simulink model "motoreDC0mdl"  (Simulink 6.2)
settings: Solver=ode45  StartTime=0.0  StopTime=10.0  RelTol=1e-6  AbsTol=1e-6
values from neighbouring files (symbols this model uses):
  bme = Ic0*KI/Wmax    (= 1.40697764938e-05)    [motoreDC0.m]
  Ime0 = 0    [motoreDC0.m]
  Jme = 7.06*mg*m^2    (= 7.06e-06)    [motoreDC0.m]
  KI = Cmax/Imax    (= 0.0452697095436)    [motoreDC0.m]
  Lme = 2.63*mHenry    (= 0.00263)    [motoreDC0.m]
  Rme0 = Vn/Imax    (= 2.48962655602)    [motoreDC0.m]
  Tcsim = 1*msec    (= 0.001)    [motoreDC0.m]
  th0 = 0    [motoreDC0.m]
  Wme0 = 0    [motoreDC0.m]
libraries: simulink x2

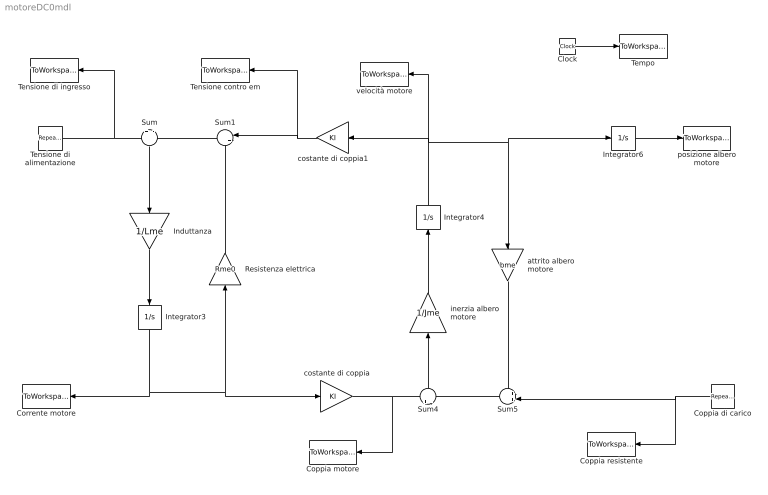
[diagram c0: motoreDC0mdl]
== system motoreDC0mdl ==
  Clock : Clock
  Coppia motore : ToWorkspace  VariableName=Cm  SampleTime=Tcsim  SaveFormat=Array
  Coppia resistente : ToWorkspace  VariableName=Cr  SampleTime=Tcsim  SaveFormat=Array
  Coppia di carico : simulink/Sources/Repeating Sequence  Orientation=left  rep_seq_t=TABTEMPI  rep_seq_y=TABCR
  Corrente motore : ToWorkspace  VariableName=Ime  SampleTime=Tcsim  SaveFormat=Array
  Induttanza : Gain  Orientation=down  Gain=1/Lme
  Integrator3 : Integrator  Orientation=down  InitialCondition=Ime0
  Integrator4 : Integrator  Orientation=up  InitialCondition=Wme0
  Integrator6 : Integrator  InitialCondition=th0
  Resistenza elettrica : Gain  Orientation=up  Gain=Rme0
  Sum : Sum  Orientation=down  Inputs=+|-
  Sum1 : Sum  Orientation=left  Inputs=|++
  Sum4 : Sum  Orientation=up  Inputs=+|-
  Sum5 : Sum  Orientation=left  Inputs=++|
  Tempo : ToWorkspace  VariableName=t  SampleTime=Tcsim  SaveFormat=Array
  Tensione contro em : ToWorkspace  VariableName=Vcem  SampleTime=Tcsim  SaveFormat=Array
  Tensione di ingresso : ToWorkspace  VariableName=Vi  SampleTime=Tcsim  SaveFormat=Array
  Tensione di alimentazione : simulink/Sources/Repeating Sequence  rep_seq_t=TABTEMPI  rep_seq_y=TABVIN
  attrito albero motore : Gain  Orientation=down  Gain=bme
  costante di coppia : Gain  Gain=KI
  costante di coppia1 : Gain  Orientation=left  Gain=KI
  inerzia albero motore : Gain  Orientation=up  Gain=1/Jme
  posizione albero motore : ToWorkspace  VariableName=th  SampleTime=Tcsim  SaveFormat=Array
  velocità motore : ToWorkspace  VariableName=Wme  SampleTime=Tcsim  SaveFormat=Array
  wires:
  Tensione di alimentazione/1 -> Sum/1, Tensione di ingresso/1
  Sum/1 -> Induttanza/1
  Induttanza/1 -> Integrator3/1
  Sum1/1 -> Sum/2
  Integrator3/1 -> Corrente motore/1, costante di coppia/1, Resistenza elettrica/1
  Resistenza elettrica/1 -> Sum1/2
  Sum4/1 -> inerzia albero motore/1
  inerzia albero motore/1 -> Integrator4/1
  Sum5/1 -> Sum4/2
  attrito albero motore/1 -> Sum5/1
  Coppia di carico/1 -> Coppia resistente/1, Sum5/2
  Integrator4/1 -> velocità motore/1, attrito albero motore/1, Integrator6/1, costante di coppia1/1
  Integrator6/1 -> posizione albero motore/1
  costante di coppia/1 -> Sum4/1, Coppia motore/1
  costante di coppia1/1 -> Sum1/1, Tensione contro em/1
  Clock/1 -> Tempo/1
